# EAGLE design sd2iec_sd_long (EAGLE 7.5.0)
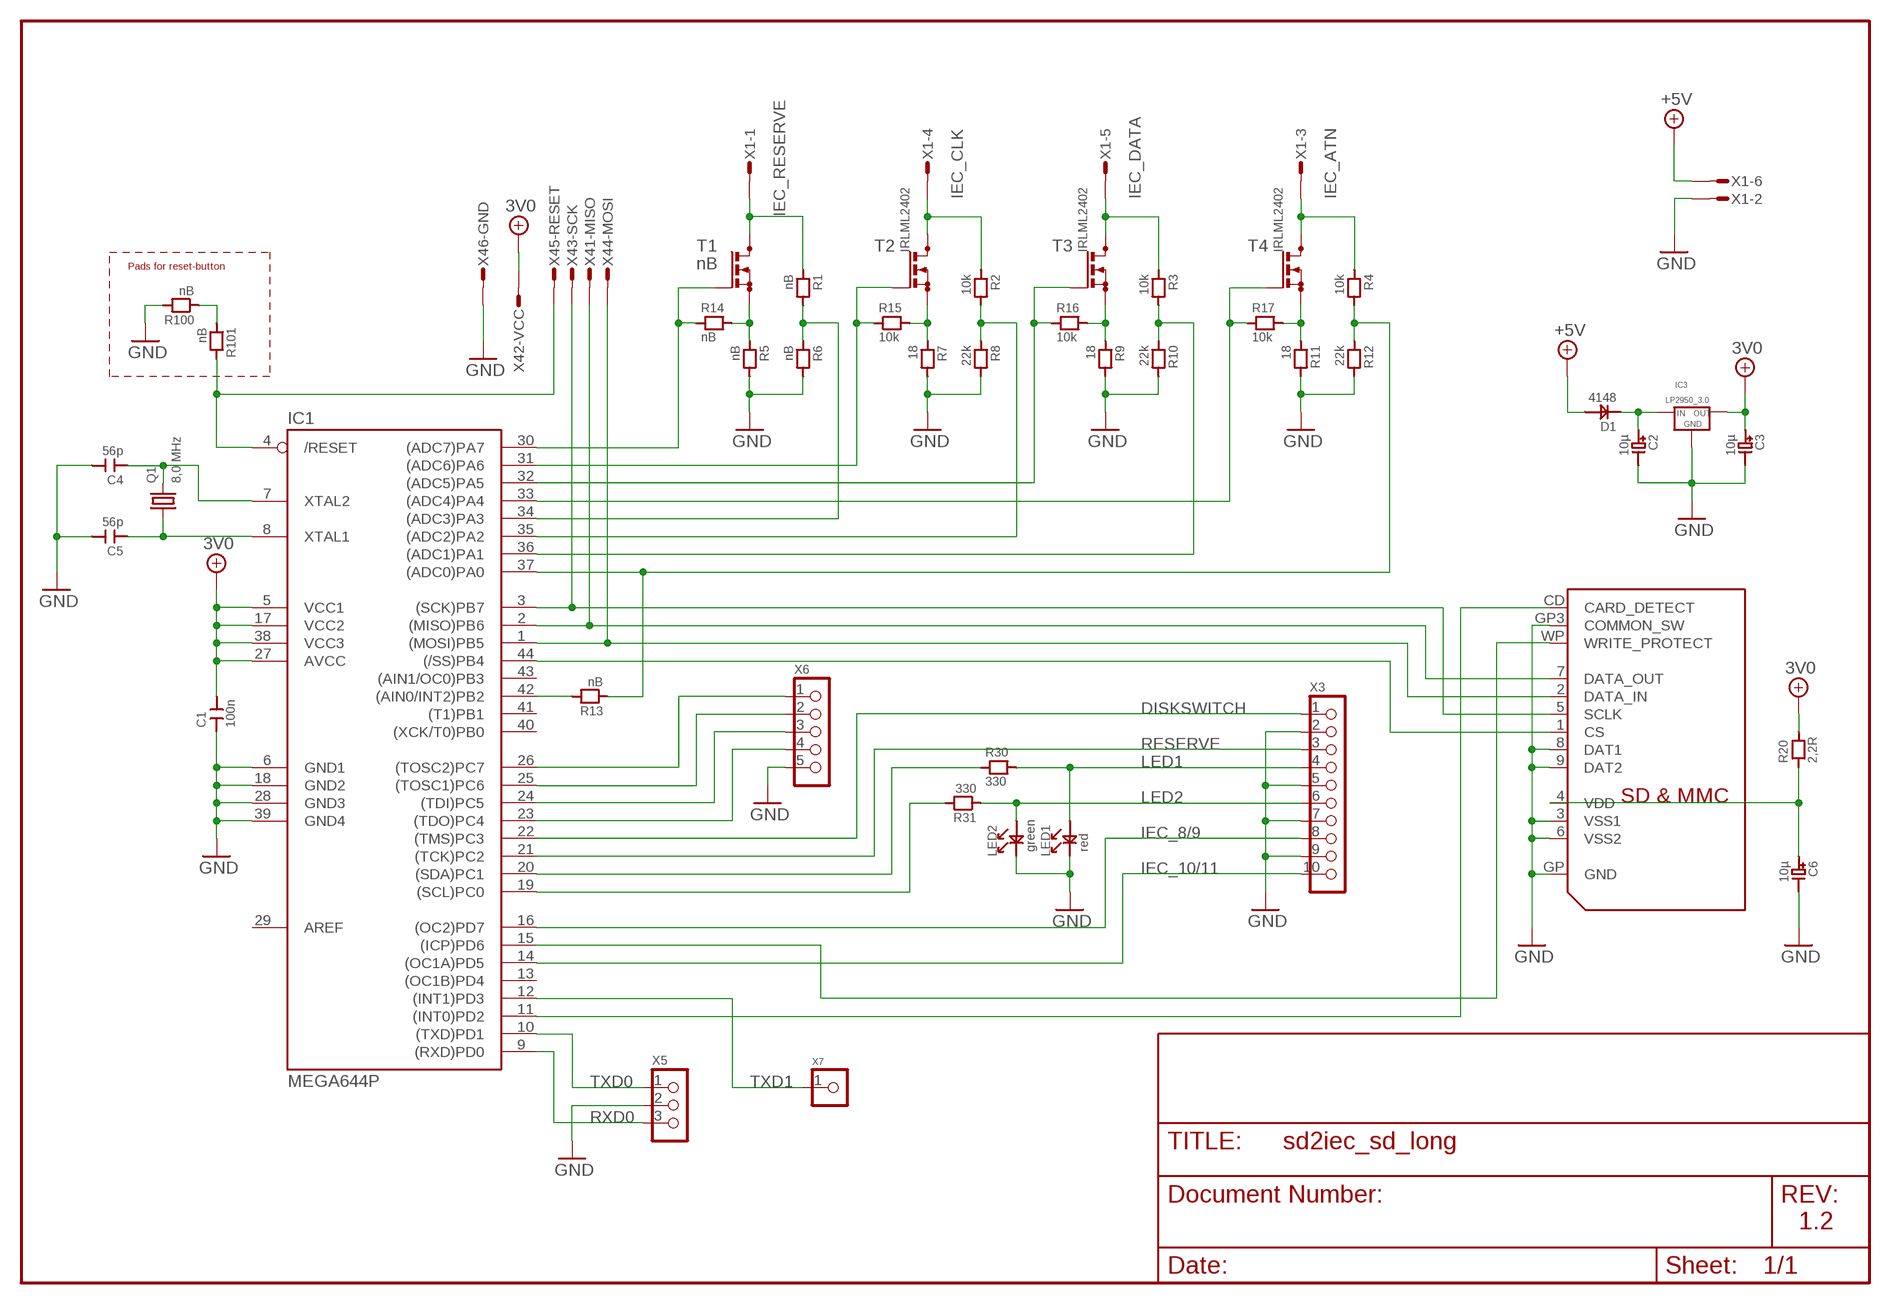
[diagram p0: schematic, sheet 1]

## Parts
C1  100n  C1206  [C1206]
C2  10µ  C_POLTA_A  [C_TANTAL_A]
C3  10µ  C_POLTA_A  [C_TANTAL_A]
C4  56p  C1206  [C1206]
C5  56p  C1206  [C1206]
C6  10µ  C_POLTA_A  [C_TANTAL_A]
D1  4148  DSOD-123  [SOD-123]
IC1  MEGA644P  MEGA16/32TQFP  [TQFP44]
IC3  LP2950_3.0  LP2950_TO92S  [TO92_S]
LED1  red  LED1206  [LED1206]
LED2  green  LED1206  [LED1206]
Q1  8,0 MHz  HC49  [HC49/S]
R1  nB  R1206  [R1206]
R2  10k  R1206  [R1206]
R3  10k  R1206  [R1206]
R4  10k  R1206  [R1206]
R5  nB  R1206  [R1206]
R6  nB  R1206  [R1206]
R7  18  R1206  [R1206]
R8  22k  R1206  [R1206]
R9  18  R1206  [R1206]
R10  22k  R1206  [R1206]
R11  18  R1206  [R1206]
R12  22k  R1206  [R1206]
R13  nB  R0603  [R0603]
R14  nB  R0805  [R0805]
R15  10k  R0805  [R0805]
R16  10k  R0805  [R0805]
R17  10k  R0805  [R0805]
R20  2,2R  R1206  [R1206]
R30  330  R1206  [R1206]
R31  330  R1206  [R1206]
R100  nB  R1206  [R1206]
R101  nB  R1206  [R1206]
T1  nB  BSN20_C  [SOT23_C]
T2  IRLML2402  BSN20_C  [SOT23_C]
T3  IRLML2402  BSN20_C  [SOT23_C]
T4  IRLML2402  BSN20_C  [SOT23_C]
U$6  SDMMC06132  [06132]
X1  MICROMATCH-6_PIN  [MICROMATCH-6]
X3  PINH1X10  [1X10]
X4  AVR-ISP_1X6  [1X6_ISP]
X5  PINH1X3  [1X3]
X6  PINH1X52,54  [1X5]
X7  PINH1X1  [1X1]

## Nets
3V0: C1.2 C3.1 IC1.5(VCC1) IC1.17(VCC2) IC1.27(AVCC) IC1.38(VCC3) IC3.3(OUT) R20.2 X4.2
+5V: D1.2 X1.6
/RESET: IC1.4(/RESET) R101.2 X4.5
ATN: IC1.37((ADC0)PA0) R4.2 R12.1 R13.1
CD: IC1.11((INT0)PD2) U$6.CD(CARD_DETECT)
CLK: IC1.35((ADC2)PA2) R2.2 R8.1
CS: IC1.44((/SS)PB4) U$6.1(CS)
DATA: IC1.36((ADC1)PA1) R3.2 R10.1
DISKSWITCH: IC1.22((TMS)PC3) X3.1
GND: C1.1 C2.2 C3.2 C4.2 C5.2 C6.2 IC1.6(GND1) IC1.18(GND2) IC1.28(GND3) IC1.39(GND4) IC3.2(GND) LED1.1 LED2.1 R5.2 R6.2 R7.2 R8.2 R9.2 R10.2 R11.2 R12.2 R100.2 U$6.3(VSS1) U$6.6(VSS2) U$6.8(DAT1) U$6.9(DAT2) U$6.GP3(COMMON_SW) U$6.GP(GND) X1.2 X3.2 X3.5 X3.7 X3.9 X4.6 X5.2 X6.5
IEC_8/9: IC1.16((OC2)PD7) X3.8
IEC_10/11: IC1.14((OC1A)PD5) X3.10
IEC_ATN: R4.1 T4.3(D) X1.3
IEC_CLK: R2.1 T2.3(D) X1.4
IEC_DATA: R3.1 T3.3(D) X1.5
IEC_RESERVE: R1.1 T1.3(D) X1.1
IECRESERVE: IC1.34((ADC3)PA3) R1.2 R6.1
LED1: LED1.2 R30.2 X3.4
LED2: LED2.2 R31.1 X3.6
MISO: IC1.2((MISO)PB6) U$6.7(DATA_OUT) X4.1
MOSI: IC1.1((MOSI)PB5) U$6.2(DATA_IN) X4.4
N$1: IC1.23((TDO)PC4) X6.4
N$2: C2.1 D1.1 IC3.1(IN)
N$3: IC1.42((AIN0/INT2)PB2) R13.2
N$4: C5.1 IC1.8(XTAL1) Q1.1
N$5: C4.1 IC1.7(XTAL2) Q1.2
N$7: IC1.24((TDI)PC5) X6.3
N$11: IC1.25((TOSC1)PC6) X6.2
N$12: IC1.26((TOSC2)PC7) X6.1
N$17: IC1.32((ADC5)PA5) R16.1 T3.1(G)
N$18: R100.1 R101.1
N$19: IC1.33((ADC4)PA4) R17.1 T4.1(G)
N$20: IC1.31((ADC6)PA6) R15.1 T2.1(G)
N$21: IC1.30((ADC7)PA7) R14.1 T1.1(G)
N$22: R5.1 R14.2 T1.2(S)
N$23: R7.1 R15.2 T2.2(S)
N$24: R9.1 R16.2 T3.2(S)
N$25: R11.1 R17.2 T4.2(S)
PC0: IC1.19((SCL)PC0) R31.2
PC1: IC1.20((SDA)PC1) R30.1
RESERVE: IC1.21((TCK)PC2) X3.3
RXD0: IC1.9((RXD)PD0) X5.3
SCK: IC1.3((SCK)PB7) U$6.5(SCLK) X4.3
TXD0: IC1.10((TXD)PD1) X5.1
TXD1: IC1.12((INT1)PD3) X7.1
VDD: C6.1 R20.1 U$6.4(VDD)
WP: IC1.15((ICP)PD6) U$6.WP(WRITE_PROTECT)
Unconnected: IC1.13((OC1B)PD4) IC1.29(AREF) IC1.40((XCK/T0)PB0) IC1.41((T1)PB1) IC1.43((AIN1/OC0)PB3)

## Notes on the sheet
- Pads for reset-button
- 1.2

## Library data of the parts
C1 C4 C5 = 0_rr:C
C2 C3 C6 = 0_rr:C_POL
D1 = 0_rr:D
IC1 = 0_rr:MEGA16/32: MICROCONTROLLER 16 Kbytes FLASH, 512 bytes EEPROM 1 Kbytes SRAM dual UART hardware multiplier
IC3 = 0_rr:LP2950
LED1 LED2 = 0_rr:LED
Q1 = 0_rr:HC49
R1-R17 R20 R30 R31 R100 R101 = 0_rr:R
T1-T4 = 0_rr:BSN20: N-CHANNEL MOS FET
U$6 = adafruit:SDMMC: SD MMC Card holder 4UCON part #06132 - easy to solder
X1 = 0_rr:MICROMATCH-6: MicroMaTch 6 7-215464-6 / 0-215464-6 Drawing Number C-215464 DDEController.pdf
X3 = 0_rr:PINH1X10
X4 = 0_rr:AVR-ISP: MicroMaTch 6 7-215464-6 / 0-215464-6 Drawing Number C-215464 DDEController.pdf
X5 = 0_rr:PINH1X3
X6 = 0_rr:PINH1X5
X7 = 0_rr:PINH1X1

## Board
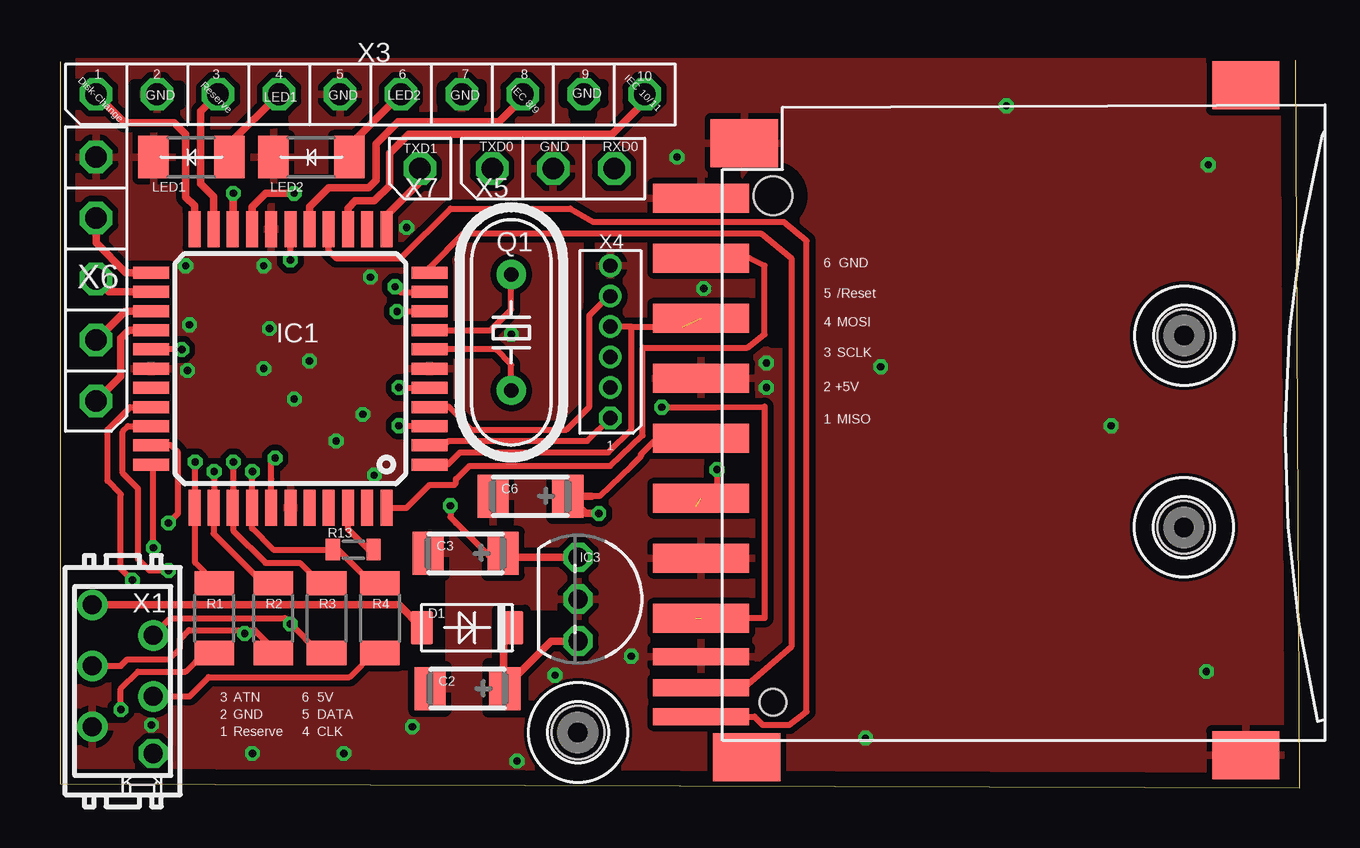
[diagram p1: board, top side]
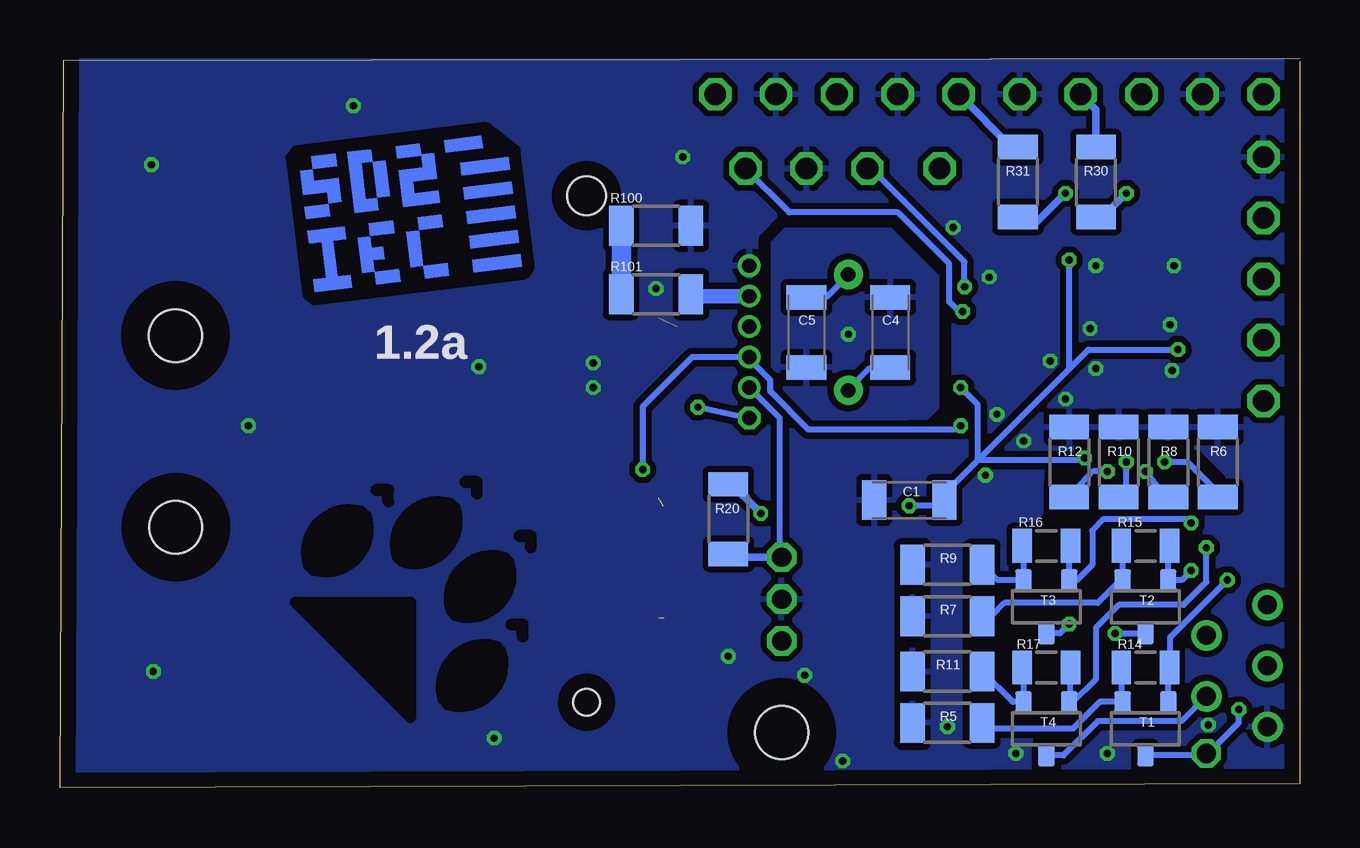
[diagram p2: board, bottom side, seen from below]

Size 51.67 x 30.32 mm. Coordinates in mm from the lower left corner, seen from the top.
Outline: 51.51,30.32 51.67,0 0,0.16 0,30.24
Copper layers (1*16): Top 0.035mm / dielectric 1.5mm / Bottom 0.035mm
Design rules "default": minimum track width 8mil, minimum drill 12mil, track to track 8mil, track to pad 8mil, pad to pad 8mil, via to via 8mil, smd to smd 8mil, copper to edge 25mil, drill to drill 8mil, minimum pad ring 6mil, minimum via ring 6mil, stop-mask expansion 4mil, vias tented up to drill 12mil, thermal gap 10mil
tRestrict: area 29.7,18.6 to 30.2,22.1; 29 lines
bRestrict: 22 lines

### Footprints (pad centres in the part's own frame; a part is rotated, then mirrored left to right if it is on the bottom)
C1206 = smd 1.016 x 1.651: 1 -1.462,0; 2 1.462,0
C_TANTAL_A = smd 1.3 x 1.8: 1 1.559,0; 2 -1.559,0
SOD-123 = smd 0.914 x 1.397: 1 -1.884,0; 2 1.884,0
TQFP44 = smd 1.5 x 0.5: 1 -5.8,4; 2 -5.8,3.2; 3 -5.8,2.4; 4 -5.8,1.6; 5 -5.8,0.8; 6 -5.8,0; 7 -5.8,-0.8; 8 -5.8,-1.6; 9 -5.8,-2.4; 10 -5.8,-3.2; 11 -5.8,-4; 23 5.8,-4; 24 5.8,-3.2; 25 5.8,-2.4; 26 5.8,-1.6; 27 5.8,-0.8; 28 5.8,0; 29 5.8,0.8; 30 5.8,1.6; 31 5.8,2.4; 32 5.8,3.2; 33 5.8,4 | smd 0.5 x 1.5: 12 -4,-5.8; 13 -3.2,-5.8; 14 -2.4,-5.8; 15 -1.6,-5.8; 16 -0.8,-5.8; 17 0,-5.8; 18 0.8,-5.8; 19 1.6,-5.8; 20 2.4,-5.8; 21 3.2,-5.8; 22 4,-5.8; 34 4,5.8; 35 3.2,5.8; 36 2.4,5.8; 37 1.6,5.8; 38 0.8,5.8; 39 0,5.8; 40 -0.8,5.8; 41 -1.6,5.8; 42 -2.4,5.8; 43 -3.2,5.8; 44 -4,5.8
TO92_S = drill 0.8 pad 1.219 octagon: 1 1.746,0; 2 0,0; 3 -1.746,0
LED1206 = smd 1.27 x 1.778: 1 -1.581,0; 2 1.581,0
HC49/S = drill 0.6 pad 1.219: 1 -2.413,0; 2 2.413,0
R1206 = smd 1.016 x 1.651: 1 -1.454,0; 2 1.454,0
R0603 = smd 0.6 x 0.9: 1 -0.85,0; 2 0.85,0
R0805 = smd 0.8 x 1.4: 1 -1.009,0; 2 1.009,0
SOT23_C = smd 0.7 x 0.9: 1 -0.953,-1.111; 2 0.953,-1.111; 3 0,1.111
2,2 = hole 2.2: 0,0
06132 = smd 1.2 x 4: 1 6.9,0.9; 2 4.4,0.9; 3 1.9,0.9; 4 -0.6,0.9; 5 -3.1,0.9; 6 -5.6,0.9; 7 -8.1,0.9; 9 9.4,0.9 | smd 0.7 x 4: 8 -9.7,0.9; CD -11,0.9; WP -12.2,0.9 | smd 2 x 2.8: GP -13.8,-21.8; GP2 14.1,-21.8; GP3 11.7,-0.9; GP4 -13.9,-1 | hole 1.1: -11.6,-2.1 | hole 1.6: 9.5,-2.1
MICROMATCH-6 = drill 0.8 pad 1.118 octagon: 1 3.016,1.27 | drill 0.8 pad 1.27: 2 1.905,-1.27; 3 0.635,1.27; 4 -0.635,-1.27; 5 -1.905,1.27; 6 -3.175,-1.27
1X10 = drill 0.9 octagon: 1 -11.43,0; 2 -8.89,0; 3 -6.35,0; 4 -3.81,0; 5 -1.27,0; 6 1.27,0; 7 3.81,0; 8 6.35,0; 9 8.89,0; 10 11.43,0
1X6_ISP = drill 0.6 pad 0.94 octagon: 1 0,0 | drill 0.6 pad 0.94: 2 1.27,0; 3 2.54,0; 4 3.81,0; 5 5.08,0; 6 6.35,0
1X3 = drill 0.9 octagon: 1 -2.54,0; 2 0,0; 3 2.54,0
1X5 = drill 0.9 octagon: 1 -5.08,0; 2 -2.54,0; 3 0,0; 4 2.54,0; 5 5.08,0
1X1 = drill 0.9 pad 1.27 octagon: 1 0,0

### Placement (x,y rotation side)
C1  16.27,11.99 0 bottom
C2  16.99,4.13 0 top
C3  16.91,9.76 0 top
C4  17.07,18.97 90 bottom
C5  20.56,18.97 270 bottom
C6  19.61,12.14 0 top
D1  16.96,6.67 180 top
IC1  9.6,17.46 180 top
IC3  21.59,7.86 270 top
LED1  5.48,26.27 0 top
LED2  10.48,26.27 0 top
Q1  18.81,18.97 270 top
R1  6.43,7.06 90 top
R2  8.89,7.06 90 top
R3  11.11,7.06 90 top
R4  13.34,7.06 90 top
R5  14.68,2.7 180 bottom
R6  3.41,13.57 90 bottom
R7  14.68,7.14 180 bottom
R8  5.48,13.57 90 bottom
R9  14.68,9.29 180 bottom
R10  7.54,13.57 90 bottom
R11  14.68,4.84 180 bottom
R12  9.6,13.57 90 bottom
R13  12.22,9.92 0 top
R14  6.43,5 180 bottom
R15  6.43,10.08 180 bottom
R16  10.56,10.08 180 bottom
R17  10.56,5 180 bottom
R20  23.81,11.19 270 bottom
R30  8.49,25.24 90 bottom
R31  11.75,25.24 270 bottom
R100  26.83,23.42 0 bottom
R101  26.83,20.56 0 bottom
T1  6.43,2.46 180 bottom
T2  6.43,7.54 180 bottom
T3  10.56,7.54 180 bottom
T4  10.56,2.46 180 bottom
U$1  [2,2]  46.86,18.84 0 top
U$2  [LOGO_B]  36.54,8.25 45 top
U$3  [2,2]  46.84,10.85 0 top
U$4  [2,2]  21.59,2.3 0 top
U$5  [SD2IEC_LOGO]  37.15,23.9 7 bottom
U$6  27.62,15.16 90 top
X1  2.62,4.44 270 top
X3  12.94,28.89 0 top
X4  22.94,15.4 90 top
X5  20.56,25.8 0 top
X6  1.51,21.19 90 top
X7  15,25.8 0 top

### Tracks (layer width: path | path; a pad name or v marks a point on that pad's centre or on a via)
3V0  (via drill 0.3)
  Top 0.254: IC1.5 v14.13,16.67 | IC1.38 8.8,11.59 8.81,11.59 8.81,12.86 8.81,13.57 v8.97,13.73 | IC1.27 v5.07,18.26 v5.08,18.26 | 18.49,9.68 18.47,9.68 17.86,9.68 16.51,11.03 16.27,11.27 v16.27,11.75 | v9.6,21.99 IC1.17
  Top 0.305: C3.1 18.47,9.68 18.55,9.6 IC3.3
  Bottom 0.254: v5.08,18.26 8.81,18.26 9.6,17.46 | 13.41,13.65 9.6,17.46 | v14.13,16.67 13.41,15.95 13.41,13.65 | X4.2 21.67,15.4 21.67,11.43 21.67,9.68 IC3.3 | v8.97,13.73 9.13,13.65 9.45,13.65 13.41,13.65 | 9.6,17.46 v9.6,21.99 | 13.41,13.65 14.81,12.26 C1.2 14.84,11.99 | 14.84,11.99 | v16.27,11.75 15.08,11.75 14.84,11.99
  Bottom 0.305: R20.2 23.81,9.61 23.81,9.6 IC3.3
+5V
  Top 0.305: X1.6 12.22,7.62 13.18,7.62 14.13,7.62 D1.2
/RESET
  Top 0.254: IC1.4 15.42,15.87 16.19,15.87 17.14,14.92 21.11,14.92 22.07,15.87 22.07,19.68 22.86,20.48 X4.5 | X4.5 | X4.5
  Bottom 0.305: 25.25,20.48 R101.2 | X4.5
  Bottom 0.61: X4.5 25.25,20.48
ATN  (via drill 0.3)
  Top 0.254: R4.2 13.02,8.49 11.59,9.92 11.27,9.92 | 11.27,9.92 8.89,9.92 8.01,10.81 IC1.37 8.02,11.67 v8.02,13.18 | 11.27,9.92 R13.1
  Bottom 0.254: R12.1 8.63,13.18 v8.02,13.18
CD
  Top 0.254: IC1.11 15.4,21.67 16.83,23.1 29.21,23.1 30.48,22.07 30.48,5.87 28.65,4.29 26.77,4.21 U$6.CD
CLK  (via drill 0.3)
  Top 0.254: R2.2 8.41,8.57 7.62,9.37 6.4,10.58 IC1.35 6.5,11.66 6.43,11.67 v6.43,13.18
  Bottom 0.254: R8.1 5.48,11.99 v6.43,13.18
CS
  Top 0.254: IC1.44 14.44,11.66 15.4,12.62 16.43,12.62 16.51,12.7 16.51,12.86 17.07,13.41 22.94,13.41 24.29,14.68 24.29,18.34 28.65,18.34 29.37,18.89 29.37,21.75 28.73,22.07 26.49,22.07 U$6.1
DATA  (via drill 0.3)
  Top 0.254: v7.22,13.57 7.22,11.68 IC1.36 7.22,11.67 7.22,10.72 8.57,9.37 10,9.37 10.85,8.52 R3.2
  Bottom 0.254: R10.1 7.22,12.07 v7.22,13.57
DISKSWITCH
  Top 0.254: X3.1
  Top 0.305: IC1.22 5.6,24.24 5.24,24.61 5.24,27.23 4.76,27.7 2.7,27.7 X3.1
GND  (via drill 0.3)
  other vias: 25.72,26.27 33.58,2.06 47.86,25.96 39.45,28.42 20.64,4.68 13.1,13.02 5.24,21.75 12.94,21.27 5.32,17.38 29.45,16.67 26.83,20.8 34.21,17.54 14.45,23.34 11.51,14.45 43.82,15.08 18.81,18.89 47.78,4.84 23.81,5.48 19.05,1.11 14.68,2.54 8.02,1.43 3.81,2.62 11.83,1.43 12.62,15.56 8.73,19.13 8.49,21.75 5.4,19.29 10.4,17.78 9.76,16.19 8.49,17.46 29.45,17.7
  pour Top (isolate 0.254): 0,0.16 0,30.24 51.59,30.24 51.59,0.08
  pour Bottom (isolate 0.254): 0,0.16 0,30.24 51.51,30.24 51.59,0.16
IEC_8/9
  Top 0.305: IC1.16 10.4,24.22 11.19,25 12.86,25 13.18,25.32 13.18,26.83 14.1,27.76 18.31,27.76 19.29,28.73 X3.8 | X3.8
IEC_10/11
  Top 0.305: IC1.14 12.01,24.15 12.3,24.45 13.1,24.45 13.73,25.08 13.73,26.43 14.53,27.23 23.02,27.23 24.37,28.57 X3.10 | X3.10
IEC_ATN
  Top 0.254: X1.3 5.4,3.81 6.19,4.6 12.06,4.6 13.1,5.64 13.26,5.64 R4.1
  Bottom 0.254: T4.3 9.84,1.35 8.41,2.78 4.92,2.78 X1.3 | X1.3 | X1.3
IEC_CLK  (via drill 0.3)
  Top 0.254: X1.4 2.54,5.08 2.8,5.34 4.55,5.34 5,5.79 5,6.19 5.37,6.56 7.7,6.56 | R2.1 8.89,5.79 8.12,6.56 7.7,6.56 | 7.7,6.56 v7.7,6.43
  Bottom 0.254: v7.7,6.43 T2.3
IEC_DATA  (via drill 0.3)
  Top 0.254: X1.5 4.6,7.06 9.37,7.06 v9.6,6.83 | v9.6,6.83 | R3.1 10.82,5.61 v9.6,6.83
  Bottom 0.254: T3.3 10,6.43 v9.6,6.83
IEC_RESERVE  (via drill 0.3)
  Top 0.254: R1.1 6.04,5.64 5.24,4.84 3.25,4.84 2.54,4.13 v2.54,3.25
  Bottom 0.254: 3.81,1.43 | X1.1 3.81,1.43 | 3.81,1.43 2.54,2.7 v2.54,3.25 2.54,3.17 | X1.1 | T1.3 3.97,1.35 X1.1
IECRESERVE  (via drill 0.3)
  Top 0.254: R1.2 6.44,8.57 5.64,9.37 5.64,11.67 | 5.64,11.67 5.64,11.75 5.6,11.72 IC1.34 5.64,11.67 | 5.64,11.67 v5.64,13.57
  Bottom 0.254: R6.1 3.41,12.3 4.68,13.57 v5.64,13.57
LED1
  Top 0.305: X3.4 | LED1.2 7.06,26.82 X3.4
  Bottom 0.305: X3.4 | R30.2 8.49,28.26 X3.4
LED2
  Top 0.305: X3.6 | LED2.2 12.06,26.74 X3.6
  Bottom 0.305: X3.6 | R31.1 12.01,26.69 X3.6
MISO  (via drill 0.3)  (1 unrouted)
  Top 0.254: IC1.2 15.43,14.29 16.03,14.29 16.19,14.45 21.99,14.45 X4.1 | X4.1 | X4.1 | 26.5,7.05 29.37,7.06 29.37,15.87 27.33,15.85 v25.08,15.85
  Bottom 0.254: X4.1 22.94,15.37 v25.08,15.85 | X4.1
MOSI  (1 unrouted)
  Top 0.254: X4.4 | 23.81,19.21 X4.4 | 23.81,19.21 25.96,19.21 | 25.96,19.21 25.98,19.21 | IC1.1 16.16,13.46 16.67,13.97 22.86,13.97 23.81,14.92 23.81,19.21 | 25.96,19.21 25.96,19.22
N$1
  Top 0.305: IC1.23 2.75,21.46 1.51,22.7 X6.4 | X6.4 | X6.4 1.51,23.81
N$2
  Top 0.305: D1.1 18.49,6.31 18.49,4.13 | C2.1 18.49,4.13 | IC3.1 20.48,6.11 18.49,4.13
N$3
  Top 0.254: R13.2 12.86,9.92 12.01,10.78 IC1.42
N$4
  Top 0.254: IC1.8 17.95,19.06 18.81,19.92 Q1.1 18.81,21.43
  Bottom 0.254: Q1.1 18.81,21.35 19.69,20.47 C5.1
N$5
  Top 0.254: IC1.7 18.17,18.26 18.81,17.62 Q1.2
  Bottom 0.254: Q1.2 18.81,16.59 17.93,17.47 C4.1
N$7
  Top 0.305: X6.3 2.04,20.66 IC1.24
N$11
  Top 0.305: X6.2 | IC1.25 2.72,19.86 X6.2
N$12
  Top 0.305: IC1.26 2.87,19.06 2.54,18.73 2.54,17.14 X6.1 | X6.1
N$17  (via drill 0.3)
  Top 0.254: IC1.32 4.63,14.26 4.92,13.97 4.92,11.43 v4.52,11.03 | v4.52,11.03
  Bottom 0.254: v4.52,11.03 | v4.52,11.03 4.68,11.19 8.18,11.19 8.65,10.72 8.65,9.29 9.29,8.65 T3.1 | T3.1 | R16.1 9.6,10.02 T3.1
N$18
  Bottom 0.813: R101.1 28.26,20.56 28.26,23.42 R100.1
N$19  (via drill 0.3)
  Top 0.254: IC1.33 3.89,13.54 v3.89,10
  Bottom 0.254: v3.89,10 3.89,8.57 4.84,7.62 7.54,7.62 8.49,6.67 8.49,4.52 9.45,3.57 9.53,3.57 | 9.53,3.57 T4.1 | R17.1 9.55,3.59 9.53,3.57
N$20  (via drill 0.3)
  Top 0.254: IC1.31 2.84,15.06 2.62,14.84 2.62,13.1 3.25,12.46 3.25,9.52 3.73,9.05 v4.52,9.05
  Bottom 0.254: v4.52,9.05 4.92,8.65 T2.1 | T2.1 | T2.1 | R15.1 5.48,10.02 T2.1
N$21  (via drill 0.3)
  Top 0.254: IC1.30 2.92,15.86 1.98,14.92 1.98,12.78 2.54,12.22 2.54,9.13 v3.02,8.65
  Bottom 0.254: v3.02,8.65 3.41,8.25 5.4,6.27 5.4,5 R14.1 5.42,4.9 5.48,4.84 T1.1
N$22
  Bottom 0.254: 7.44,3.52 T1.2 8.34,3.57 9.45,2.46 13.18,2.46 13.23,2.51 R5.1 | R14.2 7.44,3.52 | 7.44,3.52 7.46,3.49
N$23
  Bottom 0.254: R7.1 12.86,7.14 12.3,7.7 8.41,7.7 7.38,8.73 7.38,8.97 T2.2 7.38,10.02 R15.2
N$24
  Bottom 0.254: R9.1 12.6,8.65 T3.2 | T3.2 | T3.2 | R16.2 11.51,10.02 T3.2
N$25
  Bottom 0.254: R11.1 11.96,3.57 T4.2 | T4.2 | T4.2 | R17.2 11.51,4.94 T4.2
PC0  (via drill 0.3)
  Top 0.305: 8.02,23.27 IC1.19 8.01,24.2 8.57,24.76 v9.76,24.76
  Bottom 0.305: R31.2 11.75,23.58 11.75,23.57 10.95,23.57 v9.76,24.76
PC1  (via drill 0.3)
  Top 0.305: IC1.20 7.22,23.28 v7.22,24.76
  Bottom 0.305: R30.1 8.41,23.58 v7.22,24.76
RESERVE
  Top 0.254: X3.3
  Top 0.305: IC1.21 6.4,24.63 5.87,25.16 5.87,28.18 X3.3
RXD0  (via drill 0.3)
  Top 0.254: IC1.9 15.39,19.84 v14.05,19.84
  Bottom 0.254: v14.05,19.84 14.21,19.84 14.61,20.24 14.61,21.83 16.75,23.97 21.27,23.97 X5.3
SCK  (via drill 0.3)  (1 unrouted)
  Top 0.254: v27.38,13.26 27.38,12.46 26.59,11.67 26.51,11.72 | IC1.3 15.39,15.08 v14.13,15.08
  Bottom 0.254: X4.3 | X4.3 | v14.13,15.08 14.29,14.92 20.48,14.92 22.07,16.51 22.07,16.99 22.94,17.86 X4.3 | X4.3 | v27.38,13.26 27.38,15.87 25.32,17.94 X4.3 | X4.3 | X4.3
TXD0  (via drill 0.3)
  Top 0.254: IC1.10 15.38,20.64 14.21,20.64 v13.97,20.88
  Bottom 0.254: v13.97,20.88 13.97,21.91 16.75,24.69 17.86,25.8 X5.1
TXD1
  Top 0.305: IC1.12 13.6,23.84 15,25.24 X7.1
VDD  (via drill 0.3)
  Top 0.254: U$6.4 24.88,14.56 24.21,13.89 24.21,13.81 23.81,13.41 22.48,12.14 22.17,12.14
  Top 0.305: 22.17,12.14 C6.1 21.11,12.22 21.91,11.43 v22.46,11.43
  Bottom 0.305: R20.1 23.81,12.77 v22.46,11.43
WP
  Top 0.254: IC1.15 11.2,22.37 11.51,22.07 14.21,22.07 16.27,24.13 21.27,24.13 22.23,23.57 30.16,23.57 31.11,22.78 31.11,3.17 30.4,2.62 29.29,2.62 28.95,2.96 U$6.WP

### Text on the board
tPlace: 1 | 2 | Reserve | 3 | 4 | 5 | 6 | 7 | IEC 8/9 | 8 | GND | 9 | IEC 10/11 | 10 | Disk-Change | GND | LED1 | GND | LED2 | GND | TXD1 | TXD0 | GND | RXD0 | 6 | GND | 5 | /Reset | 4 | MOSI | 3 | SCLK | 2 | +5V | 1 | MISO | 1 | 2 | 3 | GND | ATN | 5 | 6 | 5V | DATA | 1 | Reserve | 4 | CLK
bPlace: 1.2a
